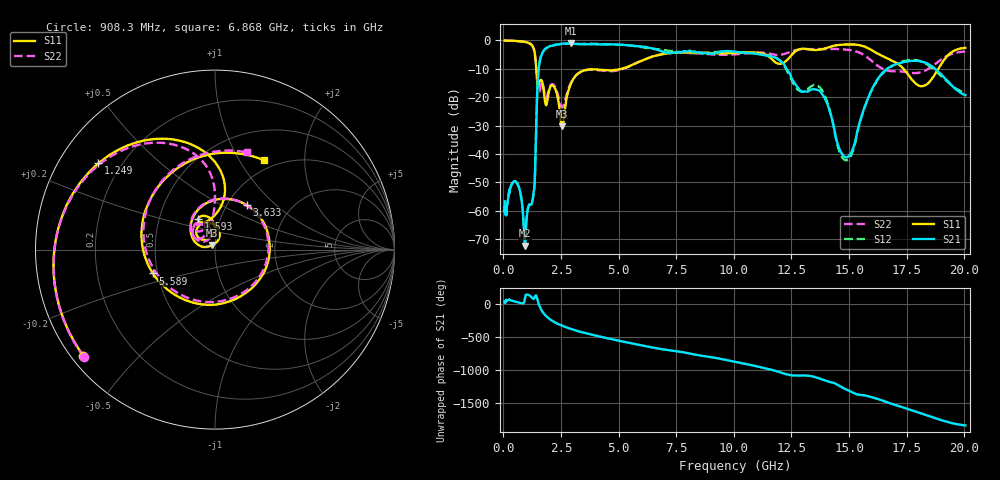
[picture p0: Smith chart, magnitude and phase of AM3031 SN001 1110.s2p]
# Hz S DB R 50
!freq MagS11 AngS11 MagS21 AngS21 MagS12 AngS12 MagS22 AngS22
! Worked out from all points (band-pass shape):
!   1601 points, 50 MHz to 20.05 GHz, reference 50 ohm
!   highest |S21| = -1.04 dB at 2.934 GHz (marker M1); lowest = -72.3 dB at 929 MHz (marker M2)
!   |S21| within 3 dB of the highest: 1.715 GHz to 6.926 GHz (5.211 GHz wide, 121 % of centre); 9.403 GHz to 10.13 GHz (722.7 MHz wide, 7.4 % of centre)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
!   lowest |S11| = -30.3 dB at 2.554 GHz (marker M3), VSWR 1.06, Z = 48.4 + j2.54 ohm
!   |S11| at or under -10 dB: 1.423 GHz to 5.136 GHz (3.714 GHz wide, 113 % of centre); 17.36 GHz to 18.87 GHz (1.51 GHz wide, 8.34 % of centre)
!   |S22| runs from -23.6 to 0.0 dB; largest |S21 - S12| = 0.067
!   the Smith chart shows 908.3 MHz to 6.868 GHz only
!   S11 on the Smith chart (normalised r, x): 908.3 MHz: 0.03, -0.35; 1.249 GHz: 0.12, +0.33; 1.593 GHz: 0.78, +0.28; 3.633 GHz: 1.23, +0.67; 5.589 GHz: 0.47, -0.15; 6.868 GHz: 0.87, +1.28
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5e7  -0.02 -7.6  -56.70 41.8  -58.27 34.4  -0.06 -7.5
1.35947e8  -0.08 -20.2  -59.11 47.1  -59.40 50.9  -0.06 -20.2
3.696318e8  -0.13 -54.6  -50.56 51.5  -50.36 52.1  -0.13 -55.2
9.083238e8  -0.52 -141.1  -70.47 40.1  -71.11 44.6  -0.50 -140.6
9.289719e8  -0.55 -144.8  -72.33 79.7  -72.49 82.1  -0.53 -144.3
1.005007e9  -0.68 -159.1  -62.67 143.2  -62.05 143.8  -0.66 -158.2
1.248914e9  -1.86 143.5  -56.89 93.0  -56.71 91.1  -1.86 145.5
1.593256e9  -14.15 118.5  -6.64 -54.7  -6.73 -54.8  -17.26 132.2
1.885814e9  -22.02 135.9  -2.58 164.5  -2.59 164.3  -19.93 142.0
2.554365e9  -30.33 120.5  -1.19 28.3  -1.22 28.5  -23.55 126.4
2.722335e9  -21.23 165.9  -1.07 5.1  -1.17 5.3  -19.68 151.3
2.934141e9  -15.15 141.1  -1.04 -20.6  -1.25 -20.1  -14.85 138.7
3.632599e9  -10.32 54.5  -1.36 -89.4  -1.16 -88.6  -10.42 59.2
5.588805e9  -8.63 -158.9  -1.84 119.2  -1.88 119.1  -8.67 -169.0
6.867543e9  -4.92 61.4  -3.84 32.6  -3.28 35.9  -4.88 71.8
7.401857e9  -4.34 10.3  -4.27 7.9  -3.94 3.7  -4.34 26.6
8.728265e9  -4.39 -105.4  -4.43 -73.2  -4.38 -71.1  -4.71 -89.8
1.021551e10  -4.37 120.7  -4.11 -171.1  -4.16 -169.9  -4.80 115.4
1.293477e10  -2.95 -104.9  -18.04 -8.0  -18.01 0.2  -3.12 -94.9
1.485787e10  -1.43 114.5  -41.25 143.4  -42.27 142.9  -3.26 129.4
1.700309e10  -7.70 -28.8  -8.48 -95.7  -8.46 -91.6  -10.90 -56.9
2.005e10  -2.61 64.1  -19.29 -47.7  -18.50 -44.4  -3.93 74.8
